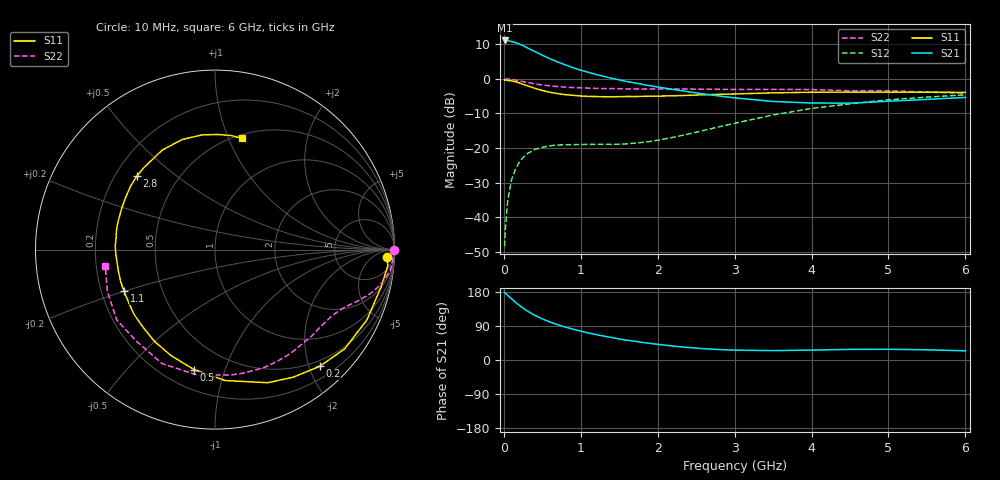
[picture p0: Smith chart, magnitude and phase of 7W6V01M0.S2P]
! Infineon Technologies  Discrete & RF Semiconductors
! BFS17W
! Si NPN RF Bipolar Junction Transistor in SOT323
! VCE = 6 V  IC = 1 mA
! Common Emitter S-Parameters:  August  1999
# GHz  S  MA  R  50
!  f  S11  S21  S12  S22
! GHz  MAG  ANG  MAG  ANG  MAG  ANG  MAG  ANG
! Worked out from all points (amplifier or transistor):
!   36 points, 10 MHz to 6 GHz, reference 50 ohm
!   highest |S21| = 11.1 dB at 10 MHz (marker M1)
!   |S21| within 3 dB of that: start of sweep to 385.4 MHz
!   unconditionally stable (mu >= 1): 1.056 GHz to end of sweep
!   at 250 MHz: K = 0.26, MSG = 16.2 dB, |S12| = -22.8 dB
!   at 1.4 GHz: K = 1.24, MAG = 6.6 dB, |S12| = -19.0 dB
!   at 6 GHz: K = 1.09, MAG = -2.2 dB, |S12| = -4.6 dB
!   S11 on the Smith chart (normalised r, x): 10 MHz: 24, -24; 200 MHz: 0.40, -2.18; 500 MHz: 0.32, -0.79; 1.1 GHz: 0.30, -0.20; 2.8 GHz: 0.29, +0.37; 6 GHz: 0.53, +1.12
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0.01  0.9588 -2.4  3.594 178.8  0.0038 84.3  0.9999 -0.2
0.02  0.9672 -5.3  3.593 176.4  0.0067 89.2  0.9878 -1.3
0.05  0.9485 -12.7  3.575 170.5  0.0172 83.0  0.9933 -3.5
0.1  0.9328 -24.8  3.461 161.6  0.0345 76.9  0.9831 -6.8
0.15  0.9095 -37.5  3.36 152.5  0.0492 68.2  0.9608 -9.8
0.2  0.8738 -48.1  3.194 144.4  0.0622 63.5  0.9378 -12.4
0.25  0.8338 -58.5  3.021 136.9  0.0727 57.3  0.9132 -14.7
0.3  0.7977 -68.4  2.833 130.1  0.0822 53.5  0.8903 -16.5
0.4  0.7315 -85.6  2.498 118.1  0.095 46.3  0.8481 -19.6
0.5  0.6784 -99.9  2.2 108.5  0.102 41.3  0.8156 -21.9
0.6  0.6395 -112.5  1.95 100.1  0.1077 37.7  0.7915 -23.9
0.7  0.6125 -123.4  1.756 93.1  0.1106 35.6  0.7734 -25.9
0.8  0.5901 -132.6  1.593 86.8  0.1113 34.2  0.7586 -27.9
1.1  0.5572 -155.6  1.243 71.2  0.1127 34.1  0.7339 -34.0
1.6  0.5561 177.9  0.914 52.3  0.1148 43.5  0.7164 -45.6
2.2  0.5692 155.5  0.704 36.7  0.1427 59.9  0.7125 -61.3
2.8  0.5976 136.6  0.565 27.6  0.2024 67.8  0.7056 -78.3
3.5  0.6276 117.9  0.471 24.8  0.3002 66.4  0.7048 -98.5
4  0.64 106.7  0.447 26.2  0.3734 60.9  0.7002 -114.8
4.5  0.6431 96.6  0.445 28.0  0.4346 54.1  0.6726 -130.2
5.5  0.6419 81.9  0.505 26.9  0.5451 40.3  0.6435 -158.8
6  0.6374 76.6  0.539 24.2  0.5873 33.8  0.6182 -171.4
